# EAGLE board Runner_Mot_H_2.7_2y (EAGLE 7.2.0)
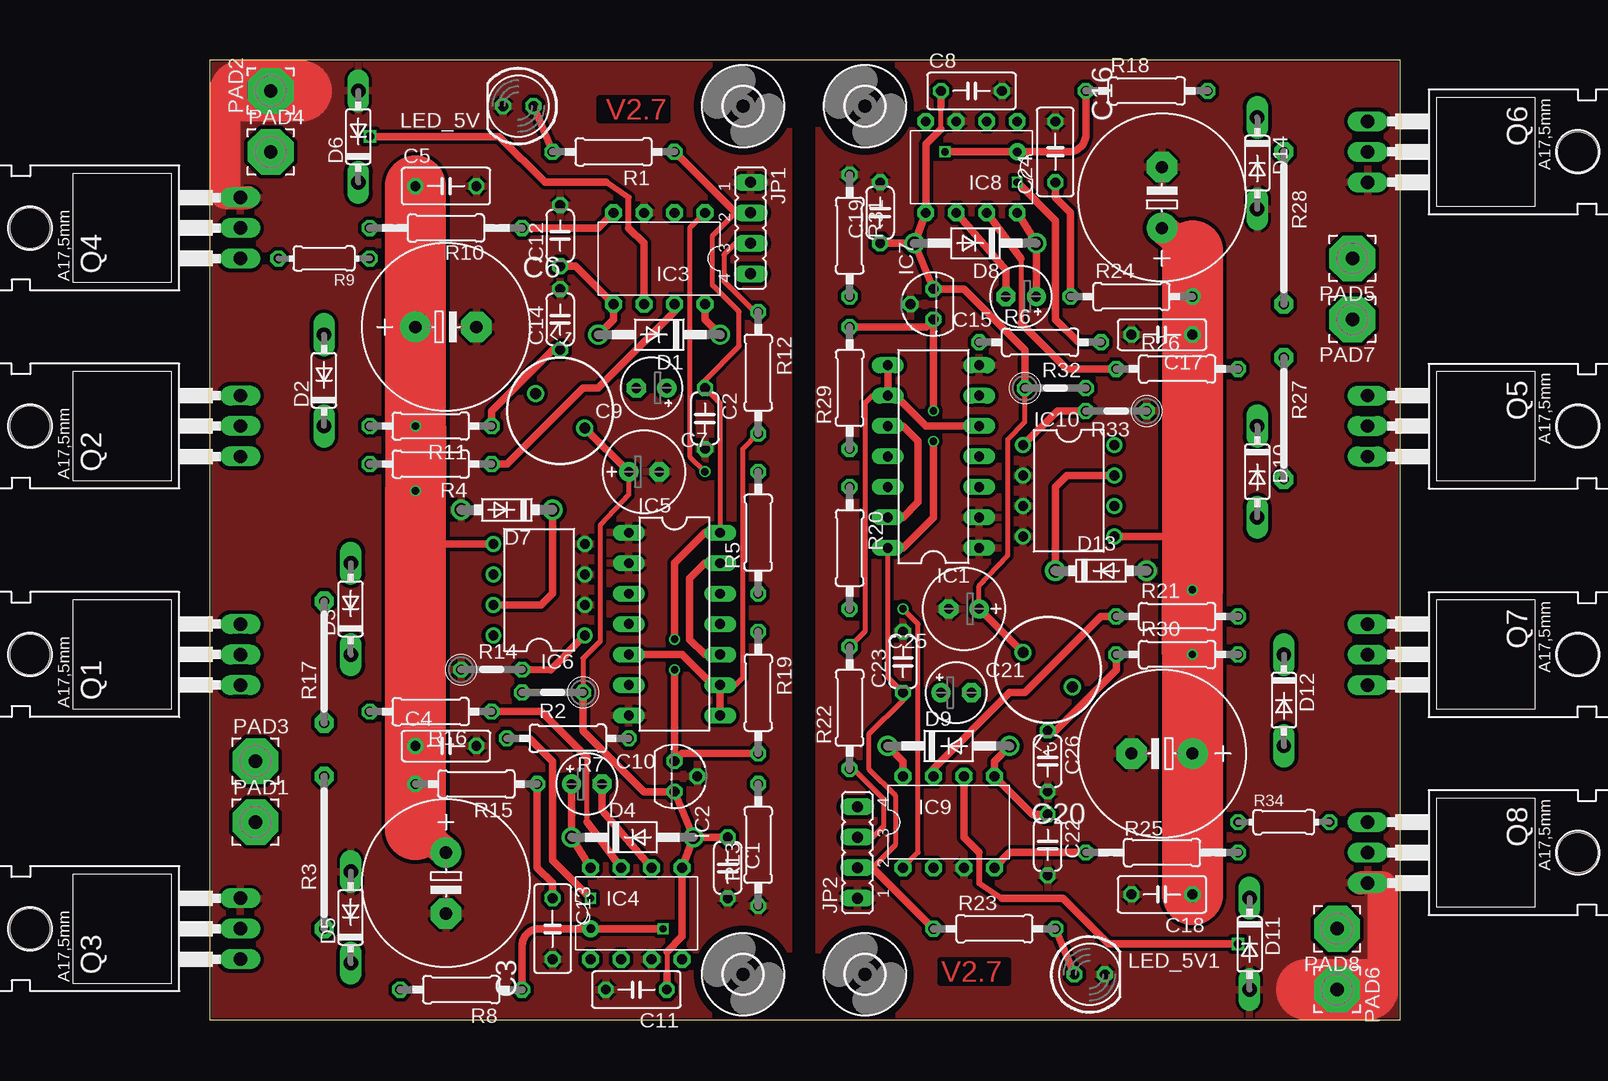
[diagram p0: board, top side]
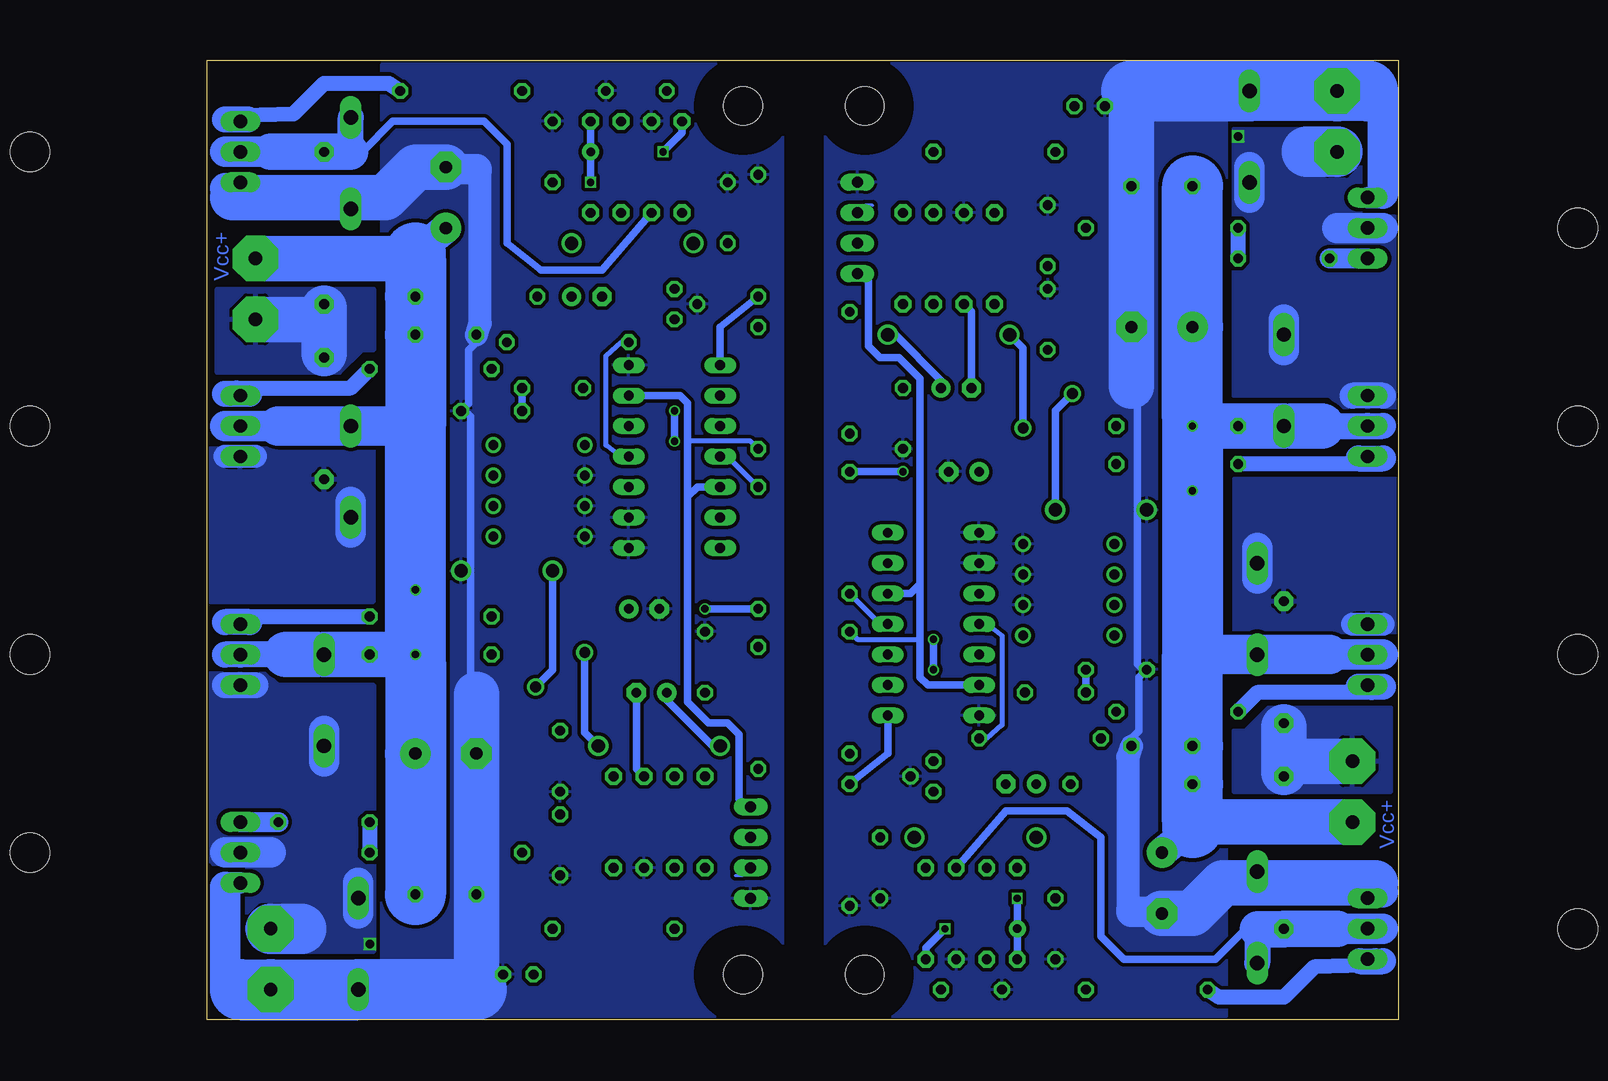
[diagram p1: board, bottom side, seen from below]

Size 99.26 x 80 mm. Coordinates in mm from the lower left corner, seen from the top.
Outline: 99.26,80 0,80 0,0 99.26,0 99.26,80
Copper layers (1*16): Top 0.035mm / dielectric 1.5mm / Bottom 0.035mm
Design rules "default *": minimum track width 6mil, minimum drill 12mil, track to track 12mil, track to pad 12mil, pad to pad 12mil, via to via 10mil, smd to smd 0mil, copper to edge 6mil, drill to drill 10mil, minimum pad ring 10mil, minimum via ring 6mil, stop-mask expansion 2mil, vias tented up to drill 100mil, thermal gap 10mil

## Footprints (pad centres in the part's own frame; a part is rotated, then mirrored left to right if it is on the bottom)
C050-024X044 = drill 0.813 octagon: 1 -2.54,0; 2 2.54,0
E5-13 = drill 1.016 pad 2.54: + -2.54,0 | drill 1.016 pad 2.54 octagon: - 2.54,0
C050-025X075 = drill 0.813 octagon: 1 -2.54,0; 2 2.54,0
C050-030X075 = drill 0.813 octagon: 1 -2.54,0; 2 2.54,0
E2,5-7 = drill 0.813 pad 1.6: + -1.27,0 | drill 0.813 pad 1.6 octagon: - 1.27,0
E2,5-5 = drill 0.813 pad 1.6: + -1.27,0 | drill 0.813 pad 1.6 octagon: - 1.27,0
DO41-10 = drill 1.118: A 5.08,0; C -5.08,0
DO35-7 = drill 1.2 long: A 3.81,0; C -3.81,0
DO41-7.6 = drill 1.1 pad 1.7: A 3.81,0; C -3.81,0
DIL14 = drill 0.813 long: 1 -7.62,-3.81; 2 -5.08,-3.81; 3 -2.54,-3.81; 4 0,-3.81; 5 2.54,-3.81; 6 5.08,-3.81; 7 7.62,-3.81; 8 7.62,3.81; 9 5.08,3.81; 10 2.54,3.81; 11 0,3.81; 12 -2.54,3.81; 13 -5.08,3.81; 14 -7.62,3.81
TO92 = drill 0.813 octagon: 1 -1.27,0; 2 0,1.905; 3 1.27,0
IRF_DIL08 = drill 0.813 pad 1.397 octagon: 1 -3.81,-3.81; 2 -1.27,-3.81; 3 1.27,-3.81; 4 3.81,-3.81; 5 3.81,3.81; 6 1.27,3.81; 7 -1.27,3.81; 8 -3.81,3.81
DIL08 = drill 0.813 pad 1.27: 1 -3.81,-3.81; 2 -1.27,-3.81; 3 1.27,-3.81; 4 3.81,-3.81; 5 3.81,3.81; 6 1.27,3.81; 7 -1.27,3.81; 8 -3.81,3.81
JP4 = drill 0.914 long: 1 -3.81,0; 2 -1.27,0; 3 1.27,0; 4 3.81,0
6000-XXXX-RC = drill 0.9 pad 1.422: 1 -2.5,0; 2 2.5,0
LED5MM = drill 0.813 octagon: A -1.27,0; K 1.27,0
3,81/1,1 = drill 1.118 pad 3.81 octagon: 1 0,0
TO220BH = drill 1.118 long: D 0,-6.35; G -2.54,-6.35; S 2.54,-6.35 | hole 3.302: 0,11.176
0207/10 = drill 0.813 octagon: 1 -5.08,0; 2 5.08,0
0207/5V = drill 0.813 octagon: 1 -2.54,0; 2 2.54,0
12 = drill 0.813 pad 1.6 octagon: 1 -6.35,0; 2 6.35,0
0204/7 = drill 0.813 octagon: 1 -3.81,0; 2 3.81,0
0207/12 = drill 0.813 octagon: 1 -6.35,0; 2 6.35,0
10 = drill 0.813 pad 1.6 octagon: 1 -5.08,0; 2 5.08,0
3,2 = hole 3.2: 0,0

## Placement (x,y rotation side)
C1  100nF  [C050-024X044]  43.18,12.69 270 top
C2  100nF  [C050-024X044]  41.27,50.16 270 top
C3  680u/50V  [E5-13]  19.68,11.42 270 top
C4  100nF  [C050-025X075]  19.68,22.85 0 top
C5  100nF  [C050-030X075]  19.68,69.52 0 top
C6  680u/50V  [E5-13]  19.68,57.77 0 top
C7  220u/16V  [E2,5-7]  36.19,45.71 0 top
C8  100nF  [C050-030X075]  63.5,77.46 0 top
C9  4u7  [E2,5-5]  36.83,52.7 180 top
C10  4u7  [E2,5-5]  31.43,19.67 0 top
C11  100nF  [C050-030X075]  35.56,2.53 180 top
C12  100nF  [C050-024X044]  29.21,65.39 90 top
C13  100nF  [C050-030X075]  28.58,7.61 270 top
C14  100nF  [C050-024X044]  29.21,58.41 90 top
C15  4u7  [E2,5-5]  67.63,60.32 180 top
C16  680u/50V  [E5-13]  79.38,68.57 90 top
C17  100nF  [C050-025X075]  79.38,57.14 180 top
C18  100nF  [C050-030X075]  79.38,10.47 180 top
C19  100nF  [C050-024X044]  55.88,67.3 90 top
C20  680u/50V  [E5-13]  79.38,22.21 180 top
C21  4u7  [E2,5-5]  62.23,27.29 0 top
C22  100nF  [C050-024X044]  69.85,14.6 270 top
C23  100nF  [C050-024X044]  57.78,29.83 90 top
C24  100nF  [C050-030X075]  70.48,72.38 90 top
C25  220u/16V  [E2,5-7]  62.87,34.28 180 top
C26  100nF  [C050-024X044]  69.85,21.58 270 top
D1  SF18G  [DO41-10]  37.47,57.14 180 top
D2  1.5KE51A  [DO35-7]  9.53,53.33 90 top
D3  1.5KE51A  [DO35-7]  11.75,34.28 90 top
D4  SF18G  [DO41-10]  35.24,15.23 0 top
D5  1.5KE51A  [DO35-7]  11.75,8.56 90 top
D6  1.5KE51A  [DO35-7]  12.38,73.65 90 top
D7  1N5819-T  [DO41-7.6]  24.77,42.54 180 top
D8  SF18G  [DO41-10]  63.82,64.76 180 top
D9  SF18G  [DO41-10]  61.59,22.85 0 top
D10  1.5KE51A  [DO35-7]  87.31,45.71 270 top
D11  1.5KE51A  [DO35-7]  86.68,6.34 270 top
D12  1.5KE51A  [DO35-7]  89.53,26.66 270 top
D13  1N5819-T  [DO41-7.6]  74.3,37.46 0 top
D14  1.5KE51A  [DO35-7]  87.31,71.43 270 top
IC1  4001N  [DIL14]  60.33,46.98 90 top
IC2  7805L  [TO92]  38.73,20.31 270 top
IC3  IRF_IR2184  [IRF_DIL08]  37.47,63.49 180 top
IC4  IRF_IR2184  [IRF_DIL08]  35.56,8.88 0 top
IC5  4001N  [DIL14]  38.73,33.01 270 top
IC6  LM2574N-ADJ  [DIL08]  27.45,35.87 90 top
IC7  7805L  [TO92]  60.33,59.68 90 top
IC8  IRF_IR2184  [IRF_DIL08]  63.5,71.11 180 top
IC9  IRF_IR2184  [IRF_DIL08]  61.59,16.5 0 top
IC10  LM2574N-ADJ  [DIL08]  71.61,44.12 270 top
JP1  PWM  [JP4]  45.09,66.03 270 top
JP2  PWM  [JP4]  53.98,13.96 90 top
L1  220uH  [6000-XXXX-RC]  29.21,50.79 325 top
L2  220uH  [6000-XXXX-RC]  69.85,29.2 145 top
LED_5V  Power  [LED5MM]  25.72,76.19 180 top
LED_5V1  Power  [LED5MM]  73.34,3.8 0 top
PAD1  36V-45V  [3,81/1,1]  3.81,16.5 0 top
PAD2  GND  [3,81/1,1]  5.08,77.46 90 top
PAD3  Motor_A  [3,81/1,1]  3.81,21.58 0 top
PAD4  Motor_B  [3,81/1,1]  5.08,72.38 0 top
PAD5  36V-45V  [3,81/1,1]  95.25,63.49 180 top
PAD6  GND  [3,81/1,1]  93.98,2.53 270 top
PAD7  Motor_A  [3,81/1,1]  95.25,58.41 180 top
PAD8  Motor_B  [3,81/1,1]  93.98,7.61 180 top
Q1  IRFB 4110  [TO220BH]  -3.81,30.47 90 top
Q2  IRFB 4110  [TO220BH]  -3.81,49.52 90 top
Q3  IRFB 4110  [TO220BH]  -3.81,7.61 90 top
Q4  IRFB 4110  [TO220BH]  -3.81,66.03 90 top
Q5  IRFB 4110  [TO220BH]  102.87,49.52 270 top
Q6  IRFB 4110  [TO220BH]  102.87,72.38 270 top
Q7  IRFB 4110  [TO220BH]  102.87,30.47 270 top
Q8  IRFB 4110  [TO220BH]  102.87,13.96 270 top
R1  1k8  [0207/10]  33.66,72.38 180 top
R2  18k  [0207/5V]  28.57,27.31 180 top
R3  0R  [12]  9.53,13.96 90 top
R4  4R7  [0207/10]  18.41,46.34 180 top
R5  4k7  [0207/10]  45.72,40.63 90 top
R6  4k7  [0207/10]  69.22,56.51 0 top
R7  4k7  [0207/10]  29.84,23.48 180 top
R8  4R7  [0207/10]  20.95,2.53 180 top
R9  4R7  [0204/7]  9.53,63.49 180 top
R10  4R7  [0207/12]  19.68,66.03 180 top
R11  0.47  [0207/10]  18.41,49.52 180 top
R12  4k7  [0207/10]  45.72,53.97 270 top
R13  100k  [0207/10]  45.72,14.6 90 top
R14  1k8  [0207/5V]  23.5,29.21 0 top
R15  0.47  [0207/10]  22.23,19.67 180 top
R16  4R7  [0207/10]  18.41,25.71 180 top
R17  0R  [10]  9.53,29.83 90 top
R18  4R7  [0207/10]  78.11,77.46 0 top
R19  100k  [0207/10]  45.72,27.29 270 top
R20  4k7  [0207/10]  53.34,39.36 270 top
R21  4R7  [0207/10]  80.64,33.65 0 top
R22  4k7  [0207/10]  53.34,26.02 90 top
R23  1k8  [0207/10]  65.41,7.61 0 top
R24  0.47  [0207/10]  76.83,60.32 0 top
R25  4R7  [0207/12]  79.38,13.96 0 top
R26  4R7  [0207/10]  80.64,54.28 0 top
R27  0R  [10]  89.53,50.16 270 top
R28  0R  [12]  89.53,66.03 270 top
R29  100k  [0207/10]  53.34,52.7 90 top
R30  0.47  [0207/10]  80.64,30.47 0 top
R31  100k  [0207/10]  53.34,65.39 270 top
R32  18k  [0207/5V]  70.48,52.68 0 top
R33  1k8  [0207/5V]  75.56,50.78 180 top
R34  4R7  [0204/7]  89.53,16.5 0 top
U$1  [3,2]  44.45,3.8 90 top
U$2  [3,2]  44.45,76.19 90 top
U$3  [3,2]  54.61,76.19 270 top
U$4  [3,2]  54.61,3.8 270 top

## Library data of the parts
C1-C26 L1 L2 R1 R2 R4-R16 R18-R26 R29-R34 = rcl
D1-D14 = diode
IC1 IC5 = 40xx
IC2 IC6 IC7 IC10 = linear
IC3 IC4 IC8 IC9 = AT3329-BTWS
JP1 JP2 R3 R17 R27 R28 = jumper
LED_5V LED_5V1 = led
PAD1-PAD8 = wirepad
Q1-Q8 = transistor-power
U$1-U$4 = holes

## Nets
GND: C1.2 C2.2 C3.- C4.2 C5.2 C6.- C7.- C11.2 C12.2 C13.2 C14.2 D5.A D6.A D7.A IC2.2 IC3.3 IC4.3 IC5.1 IC5.2 IC5.7 IC6.2 IC6.3 IC6.4 JP1.1 LED_5V.K PAD2.1 Q3.S Q4.S R13.1 R14.1
GND1: C8.2 C16.- C17.2 C18.2 C19.2 C20.- C22.2 C23.2 C24.2 C25.- C26.2 D11.A D13.A D14.A IC1.1 IC1.2 IC1.7 IC7.2 IC8.3 IC9.3 IC10.2 IC10.3 IC10.4 JP2.1 LED_5V1.K PAD6.1 Q6.S Q8.S R31.1 R33.1
N$1: IC3.1 R5.2
N$3: C10.- D5.C IC4.6 Q3.D R3.1
N$4: C10.+ D4.C IC4.8
N$5: IC4.7 R16.1
N$6: Q1.G R16.2
N$7: IC4.1 IC4.4 R7.2 R8.1
N$8: Q3.G R8.2
N$9: C9.- D2.A D6.C IC3.6 PAD4.1 Q2.S Q4.D
N$10: C9.+ D1.C IC3.8
N$11: IC3.7 R4.1
N$12: Q2.G R4.2
N$13: IC3.4 R10.1
N$14: Q4.G R9.2
N$15: C13.1 R15.1
N$16: C14.1 R11.1
N$17: IC5.4 R7.1
N$18: IC5.11 R5.1
N$19: IC5.6 IC5.12 JP1.4 R19.1
N$20: IC5.5 IC5.8 IC5.9 R12.2 R13.2
N$21: IC5.10 IC5.13
N$22: IC6.1 R2.2 R14.2
N$23: R9.1 R10.2
N$24: LED_5V.A R1.2
N$25: JP1.3 R12.1
N$27: PAD3.1 R3.2 R17.1
N$28: C15.+ D8.C IC8.8
N$29: D3.A Q1.S R17.2
N$30: IC8.7 R26.1
N$32: IC8.1 IC8.4 R6.2 R18.1
N$33: D7.C IC6.7 L1.1
N$34: Q6.G R18.2
N$35: C21.- D11.C D12.A IC9.6 PAD8.1 Q7.S Q8.D
N$36: C21.+ D9.C IC9.8
N$37: IC9.7 R21.1
N$38: Q7.G R21.2
N$39: IC1.4 R6.1
N$40: IC1.11 R20.1
N$41: IC1.6 IC1.12 JP2.4 R29.1
N$42: IC1.5 IC1.8 IC1.9 R22.2 R31.2
N$43: IC1.10 IC1.13
N$44: C15.- D14.C IC8.6 Q6.D R28.1
N$45: LED_5V1.A R23.2
N$46: IC9.1 R20.2
N$47: IC9.4 R25.1
N$48: JP2.3 R22.1
N$49: C24.1 R24.1
N$50: D10.A Q5.S R27.2
N$51: Q5.G R26.2
N$52: PAD7.1 R27.1 R28.2
N$53: C26.1 R30.1
N$54: IC10.1 R32.2 R33.2
N$55: D13.C IC10.7 L2.1
N$56: Q8.G R34.2
N$57: R25.2 R34.1
VCC1: C16.+ C17.1 C18.1 C20.+ D10.C D12.C IC10.5 PAD5.1 Q5.D Q7.D R24.2 R30.2
VCC2: C8.1 C19.1 C22.1 C25.+ D8.A D9.A IC7.3 IC8.5 IC9.5 L2.2 R32.1
VCC3: C23.1 IC1.14 IC7.1 JP2.2 R23.1 R29.2
VCC5: C2.1 IC2.1 IC5.14 JP1.2 R1.1 R19.2
VCC15: C1.1 C7.+ C11.1 C12.1 D1.A D4.A IC2.3 IC3.5 IC4.5 L1.2 R2.1
VCC24: C3.+ C4.1 C5.1 C6.+ D2.C D3.C IC6.5 PAD1.1 Q1.D Q2.D R11.2 R15.2

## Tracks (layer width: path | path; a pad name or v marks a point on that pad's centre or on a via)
GND
  Top 1.93: 1.27,68.57 3.17,68.57
  Top 2.54: 1.27,77.78 1.27,68.89
  Top 5.08: 2.54,77.46 7.62,77.46
  Bottom 0.61: 22.23,52.85 22.23,51.58 21.75,51.58 21.75,29.68 21.29,29.21 R14.1 21.59,28.58 21.59,24.12 22.23,23.48 C4.2 | 19.84,9.04 C3.-
  Bottom 1.27: 1.91,11.42 Q3.S 1.75,10.63
  Bottom 1.778: 1.75,10.63 1.91,10.63 | 1.27,68.57 Q4.S 1.91,68.57
  Bottom 1.93: C4.2 22.54,21.9 22.54,9.2 22.23,9.2 22.23,9.04
  Bottom 2.54: 1.91,10.63 1.27,10.63 | 22.23,9.04 19.84,9.04 | 1.27,68.89 1.27,77.46 2.54,77.46
  Bottom 3.81: 22.23,52.85 C6.- C5.2 22.23,77.46 | C3.- 17.14,8.88 14.61,11.42 1.91,11.42
  Bottom 5.08: 22.23,77.46 D6.A PAD2.1 2.54,77.46
  pour Bottom: 14.29,80 47.78,79.68 47.78,0.31 14.29,0.31
  pour Top: 0,-0.01 0,80 48.26,80 48.26,-0.01
GND1
  Top 1.93: 97.79,11.42 95.89,11.42
  Top 2.54: 97.79,2.21 97.79,11.1
  Top 5.08: 96.52,2.53 91.44,2.53
  Bottom 0.61: 76.83,27.14 76.83,28.41 77.31,28.41 77.31,50.31 77.78,50.78 R33.1 77.47,51.41 77.47,55.87 76.83,56.51 C17.2 | 79.22,70.95 C16.-
  Bottom 1.27: 97.16,68.57 Q6.S 97.31,69.36
  Bottom 1.778: 97.31,69.36 97.16,69.36 | 97.79,11.42 Q8.S 97.16,11.42
  Bottom 1.93: C17.2 76.52,58.09 76.52,70.79 76.83,70.79 76.83,70.95
  Bottom 2.54: 97.16,69.36 97.79,69.36 | 76.83,70.95 79.22,70.95 | 97.79,11.1 97.79,2.53 96.52,2.53
  Bottom 3.81: 76.83,27.14 C20.- C18.2 76.83,2.53 | C16.- 81.92,71.11 84.45,68.57 97.16,68.57
  Bottom 5.08: 76.83,2.53 D11.A PAD6.1 96.52,2.53
  pour Bottom: 84.77,-0.01 51.28,0.31 51.28,79.68 84.77,79.68
  pour Top: 99.06,80 99.06,-0.01 50.8,-0.01 50.8,80
N$1  (via drill 0.61)
  Top 0.406: v41.27,45.71 40.01,46.98 40.01,66.03 IC3.1
  Bottom 0.61: v41.27,45.71 R5.2
N$3
  Top 0.61: IC4.6 32.7,17.49 C10.-
  Bottom 0.152: D5.C 11.43,6.34 11.43,7.58
  Bottom 0.61: 11.68,7.58 12.73,7.58 15.24,5.07 22.86,5.07 24.77,6.98 24.77,15.23 27.62,17.45 32.7,17.45 IC4.6
  Bottom 2.184: 11.75,7.61 D5.C
  Bottom 2.54: 1.27,7.61 Q3.D 5.08,7.61
  Bottom 3.048: 5.08,7.61 R3.1 9.53,7.58 11.43,7.58 11.68,7.58
N$4
  Top 0.61: IC4.8 D4.C C10.+
N$5
  Top 0.406: 31.43,16.5 31.43,21.9
  Top 0.61: R16.1 27.62,25.71 31.43,21.9 | IC4.7 31.43,16.5
N$6
  Bottom 1.27: Q1.G 3.3,27.77 2.22,27.29 11.75,27.29 R16.2
  Bottom 2.184: 1.27,27.77 3.3,27.77
N$7  (via drill 0.6, 0.7 pad 1.42)
  Top 0.61: R8.1 26.04,6.19 arc-90 27.45,7.61 v31.75,7.61 v37.78,7.61 | R7.2 26.67,23.48 28.57,21.58 28.57,13.33 v31.75,10.15
  Bottom 0.61: v37.78,7.61 39.37,6.02 IC4.4 | IC4.1 v31.75,7.61 v31.75,10.15
N$8
  Bottom 0.152: 1.91,4.91 1.91,5.07 Q3.G
  Bottom 1.27: Q3.G 2.69,4.57 6.99,4.44 9.53,1.9 14.92,1.9 R8.2
  Bottom 2.184: 3.17,4.91 1.91,4.91 1.27,4.91
N$9  (via drill 0.7)
  Top 0.508: 34.92,66.03 34.92,68.57 33.02,69.84
  Top 0.61: 33.02,69.84 27.94,69.84 24.13,73.65 v13.34,73.65 | 34.92,66.03 36.2,64.76 IC3.6
  Bottom 0.61: C9.- 35.56,59.05 IC3.6
  Bottom 2.184: 1.27,52.06 3.81,52.06 | 1.27,66.03 3.81,66.03
  Bottom 2.54: 5.08,66.03 1.27,66.03 | 9.53,55.87 9.53,58.41 | 12.38,68.57 12.38,71.11
  Bottom 4.216: 7.62,72.38 PAD4.1
  pour Bottom: 0,51.11 4.6,51.11 5.71,52.06 13.65,52.06 13.65,74.28 3.81,74.28 3.17,73.65 3.17,66.98 0.32,66.98 0,66.66
N$10
  Top 0.61: IC3.8 41.27,58.41 D1.C
  Bottom 0.61: C9.+ 38.1,53.33 41.91,57.14 D1.C | C9.+
N$11
  Top 0.61: IC3.7 38.73,59.05 32.38,52.7 31.11,52.7 24.77,46.34 R4.1
N$12
  Bottom 0.457: Q2.G 1.43,46.98 3.3,46.82
  Bottom 1.27: Q2.G 2.54,46.34 R4.2
  Bottom 2.184: 3.3,46.82 1.27,46.82
N$13
  Top 0.61: R10.1 32.38,66.03 IC3.4
N$14
  Bottom 1.676: Q4.G R9.2
N$15
  Top 0.61: R15.1 27.3,12.69 28.57,11.42 C13.1
N$16
  Top 0.61: R11.1 23.5,50.79 28.57,55.87 C14.1
N$17
  Bottom 0.406: 34.29,33.01 33.02,32.06 33.02,24.6 34.29,23.48 R7.1
  Bottom 0.61: IC5.4 34.29,33.01
N$18
  Bottom 0.406: IC5.11 43.18,33.01 R5.1
N$19
  Bottom 0.406: 44.13,61.59 JP1.4 | R19.1 45.09,31.74 39.85,31.74
  Bottom 0.61: 44.13,61.59 44.13,56.19 43.18,55.23 41.59,55.23 39.85,53.49 39.85,36.34 | 39.85,36.34 40.64,35.55 IC5.12 43.18,35.55 | IC5.6 39.21,27.93 39.85,28.56 39.85,31.74 39.85,36.34
N$20
  Top 0.406: R12.2 44.45,47.62 44.45,28.56 43.81,27.93 IC5.9
  Top 0.61: IC5.8 IC5.9 41.91,27.93 39.37,30.47 IC5.5
  Bottom 0.61: R13.2 42.55,22.21 IC5.8
N$21
  Top 0.61: IC5.10 41.27,30.47 40.01,31.74 40.01,36.82 41.27,38.09 IC5.13
N$22
  Top 0.61: IC6.1 28.4,29.2 R14.2
  Bottom 0.254: R14.2
  Bottom 0.61: R14.2 R2.2
N$23
  Bottom 1.27: R9.1 R10.2
N$24
  Top 0.61: LED_5V.A R1.2
N$25
  Top 0.406: R12.1 45.4,59.05 42.86,61.59 42.86,63.81 43.81,64.76 JP1.3
N$27
  Bottom 0.152: R3.2 9.53,20.63 | 9.53,22.85 9.21,21.58 | R17.1 9.53,24.44
  Bottom 3.81: PAD3.1 9.21,21.58 | 9.53,20.63 9.53,22.85 9.53,24.44
  pour Bottom: 13.65,19.04 13.65,24.12 12.7,24.12 10.79,26.02 0.64,26.02 0.64,19.04
N$28
  Top 0.61: IC8.8 D8.C C15.+
N$29
  Bottom 1.93: 3.81,33.01 1.27,33.01
  Bottom 2.54: 11.75,36.82 11.75,39.36
  pour Bottom: 13.65,45.08 13.65,32.38 0,32.38 0,45.08
N$30
  Top 0.406: 67.63,63.49 67.63,58.09
  Top 0.61: R26.1 71.44,54.28 67.63,58.09 | IC8.7 67.63,63.49
N$32  (via drill 0.6, 0.7 pad 1.42)
  Top 0.61: R18.1 73.03,73.8 arc-90 71.61,72.38 v67.31,72.38 v61.28,72.38 | R6.2 72.39,56.51 70.48,58.41 70.48,66.66 v67.31,69.84
  Bottom 0.61: v61.28,72.38 59.69,73.97 IC8.4 | IC8.1 v67.31,72.38 v67.31,69.84
N$33
  Top 0.61: D7.C 28.57,35.55 27.62,34.6 IC6.7
  Bottom 0.61: D7.C 28.57,50.81 L1.1
N$34
  Bottom 0.152: 97.16,75.08 97.16,74.92 Q6.G
  Bottom 1.27: Q6.G 96.37,75.42 92.08,75.55 89.53,78.09 84.14,78.09 R18.2
  Bottom 2.184: 95.89,75.08 97.16,75.08 97.79,75.08
N$35  (via drill 0.7)
  Top 0.508: 64.14,13.96 64.14,11.42 66.04,10.15
  Top 0.61: 66.04,10.15 71.12,10.15 74.93,6.34 v85.72,6.34 | 64.14,13.96 62.87,15.23 IC9.6
  Bottom 0.61: C21.- 63.5,20.94 IC9.6
  Bottom 2.184: 97.79,27.93 95.25,27.93 | 97.79,13.96 95.25,13.96
  Bottom 2.54: 93.98,13.96 97.79,13.96 | 89.53,24.12 89.53,21.58 | 86.68,11.42 86.68,8.88
  Bottom 4.216: 91.44,7.61 PAD8.1
  pour Bottom: 99.06,28.88 94.46,28.88 93.34,27.93 85.41,27.93 85.41,5.71 95.25,5.71 95.89,6.34 95.89,13.01 98.74,13.01 99.06,13.33
N$36
  Top 0.61: IC9.8 57.78,21.58 D9.C
  Bottom 0.61: C21.+ 60.96,26.66 57.15,22.85 D9.C | C21.+
N$37
  Top 0.61: IC9.7 60.33,20.94 66.67,27.29 67.94,27.29 74.3,33.65 R21.1
N$38
  Bottom 0.457: Q7.G 97.63,33.01 95.76,33.17
  Bottom 1.27: Q7.G 96.52,33.65 R21.2
  Bottom 2.184: 95.76,33.17 97.79,33.17
N$39
  Bottom 0.406: 64.77,46.98 66.04,47.93 66.04,55.39 64.77,56.51 R6.1
  Bottom 0.61: IC1.4 64.77,46.98
N$40
  Bottom 0.406: IC1.11 55.88,46.98 R20.1
N$41
  Bottom 0.406: 54.93,18.4 JP2.4 | R29.1 53.98,48.25 59.21,48.25
  Bottom 0.61: 54.93,18.4 54.93,23.8 55.88,24.75 57.47,24.75 59.21,26.5 59.21,43.65 | 59.21,43.65 58.42,44.44 IC1.12 55.88,44.44 | IC1.6 59.85,52.06 59.21,51.43 59.21,48.25 59.21,43.65
N$42
  Top 0.406: R22.2 54.61,32.38 54.61,51.43 55.24,52.06 IC1.9
  Top 0.61: IC1.8 IC1.9 57.15,52.06 59.69,49.52 IC1.5
  Bottom 0.61: R31.2 56.52,57.77 IC1.8
N$43
  Top 0.61: IC1.10 57.78,49.52 59.05,48.25 59.05,43.17 57.78,41.9 IC1.13
N$44
  Top 0.61: IC8.6 66.36,62.5 C15.-
  Bottom 0.152: D14.C 87.63,73.65 87.63,72.41
  Bottom 0.61: 87.38,72.41 86.33,72.41 83.82,74.92 76.2,74.92 74.3,73.02 74.3,64.76 71.44,62.54 66.36,62.54 IC8.6
  Bottom 2.184: 87.31,72.38 D14.C
  Bottom 2.54: 97.79,72.38 Q6.D 93.98,72.38
  Bottom 3.048: 93.98,72.38 R28.1 89.53,72.41 87.63,72.41 87.38,72.41
N$45
  Top 0.61: LED_5V1.A R23.2
N$46  (via drill 0.61)
  Top 0.406: v57.78,34.28 59.05,33.01 59.05,13.96 IC9.1
  Bottom 0.61: v57.78,34.28 R20.2
N$47
  Top 0.61: R25.1 66.67,13.96 IC9.4
N$48
  Top 0.406: R22.1 53.66,20.94 56.2,18.4 56.2,16.18 55.24,15.23 JP2.3
N$49
  Top 0.61: R24.1 71.75,67.3 70.48,68.57 C24.1
N$50
  Bottom 1.93: 95.25,46.98 97.79,46.98
  Bottom 2.54: 87.31,43.17 87.31,40.63
  pour Bottom: 85.41,34.91 85.41,47.62 99.06,47.62 99.06,34.91
N$51
  Bottom 1.27: Q5.G 95.76,52.22 96.84,52.7 87.31,52.7 R26.2
  Bottom 2.184: 97.79,52.22 95.76,52.22
N$52
  Bottom 0.152: R28.2 89.53,59.36 | 89.53,57.14 89.85,58.41 | R27.1 89.53,55.55
  Bottom 3.81: PAD7.1 89.85,58.41 | 89.53,59.36 89.53,57.14 89.53,55.55
  pour Bottom: 85.41,60.95 85.41,55.87 86.36,55.87 88.27,53.97 98.42,53.97 98.42,60.95
N$53
  Top 0.61: R30.1 75.56,29.2 70.48,24.12 C26.1
N$54
  Top 0.61: IC10.1 70.66,50.79 R33.2
  Bottom 0.254: R33.2
  Bottom 0.61: R33.2 R32.2
N$55
  Top 0.61: D13.C 70.48,44.44 71.44,45.39 IC10.7
  Bottom 0.61: D13.C 70.48,29.18 L2.1
N$56
  Bottom 1.676: Q8.G R34.2
N$57
  Bottom 1.27: R34.1 R25.2
VCC1  (via drill 0.61)
  Top 0.406: v81.92,35.87 80.01,35.23
  Top 0.61: 80.01,35.23 v81.91,35.87 | 81.28,64.44 81.28,64.76 81.92,64.12 | IC10.5 81.92,40.31
  Top 2.54: 81.28,64.44 C16.+
  Top 5.08: 81.92,64.12 81.92,40.31 v81.92,35.87 v81.92,30.47 C18.1
  Bottom 0.254: C18.1 81.92,10.15 | 81.92,40.63 83.19,40
  Bottom 0.406: 81.92,40.63 81.91,40.47
  Bottom 0.61: 81.91,49.36 81.92,49.52
  Bottom 2.184: 97.79,30.47 Q7.D 92.71,30.47 | D12.C 90.17,30.47
  Bottom 2.54: 81.92,63.97 C16.+ | v81.92,30.47 81.92,29.83 | 97.79,49.52 Q5.D 93.34,49.52
  Bottom 3.302: 81.92,49.52 D10.C 93.34,49.52
  Bottom 3.81: v81.92,30.47 R30.2 D12.C | PAD5.1 81.92,63.49 | 92.71,30.47 90.17,30.47
  Bottom 5.08: 81.92,63.97 81.92,63.49 R24.2 C17.1 81.92,49.52 | 81.92,29.83 C20.+ C18.1 | 81.91,49.36 81.91,40.47 81.91,35.55 | v81.92,30.47 v81.92,35.87
VCC2
  Top 0.406: 60.96,74.28 60.96,76.19 | C25.+ 64.14,36.19 66.52,38.73 66.52,48.41 67.94,49.84 R32.1
  Top 0.61: D8.A IC7.3 62.87,60.95 67.94,55.87 R32.1 | 60.96,76.19 C8.1 | 60.96,74.28 59.69,73.02 IC8.5 D8.A | D9.A 65.41,21.58 IC9.5 68.58,17.13 C22.1 | C19.1 D8.A | C25.+ 64.16,34.28 L2.2
  Bottom 0.61: L2.2 67.8,23.98 D9.A
VCC3  (via drill 0.6)
  Top 0.254: C23.1
  Top 0.406: IC1.14 56.52,28.56 C23.1 57.78,26.66 54.93,23.8 54.93,20.94 57.15,18.72 57.15,14.6 55.24,12.69
  Top 0.61: R23.1 55.24,12.69 JP2.2 | IC1.14 57.78,39.36 60.33,41.9 v60.33,48.25 | v60.33,50.79 IC7.1 59.69,57.77 R29.2
  Bottom 0.254: JP2.2 54.61,12.05 55.24,12.05
  Bottom 0.61: v60.33,48.25 v60.33,50.79
VCC5  (via drill 0.6)
  Top 0.254: C2.1
  Top 0.406: IC5.14 42.55,51.43 C2.1 41.27,53.33 44.13,56.19 44.13,59.05 41.91,61.27 41.91,65.39 43.81,67.3
  Top 0.61: R1.1 43.81,67.3 JP1.2 | IC5.14 41.27,40.63 38.73,38.09 v38.73,31.74 | v38.73,29.2 IC2.1 39.37,22.21 R19.2
  Bottom 0.254: JP1.2 44.45,67.93 43.81,67.93
  Bottom 0.61: v38.73,31.74 v38.73,29.2
VCC15
  Top 0.406: 38.1,5.71 38.1,3.8 | C7.+ 34.92,43.8 32.54,41.27 32.54,31.58 31.11,30.15 R2.1
  Top 0.61: D4.A IC2.3 36.2,19.04 31.11,24.12 R2.1 | 38.1,3.8 C11.1 | 38.1,5.71 39.37,6.98 IC4.5 D4.A | D1.A 33.66,58.41 IC3.5 30.48,62.86 C12.1 | C1.1 D4.A | C7.+ 34.91,45.71 L1.2
  Bottom 0.61: L1.2 31.26,56.01 D1.A
VCC24  (via drill 0.61)
  Top 0.406: v17.14,44.12 19.05,44.76
  Top 0.61: 19.05,44.76 v17.15,44.12 | 17.78,15.55 17.78,15.23 17.14,15.87 | IC6.5 17.14,39.68
  Top 2.54: 17.78,15.55 C3.+
  Top 5.08: 17.14,15.87 17.14,39.68 v17.14,44.12 v17.14,49.52 C5.1
  Bottom 0.254: C5.1 17.14,69.84 | 17.14,39.36 15.88,40
  Bottom 0.406: 17.14,39.36 17.15,39.52
  Bottom 0.61: 17.15,30.63 17.14,30.47
  Bottom 2.184: 1.27,49.52 Q2.D 6.35,49.52 | D2.C 8.89,49.52
  Bottom 2.54: 17.14,16.02 C3.+ | v17.14,49.52 17.14,50.16 | 1.27,30.47 Q1.D 5.71,30.47
  Bottom 3.302: 17.14,30.47 D3.C 5.71,30.47
  Bottom 3.81: v17.14,49.52 R11.2 D2.C | PAD1.1 17.14,16.5 | 6.35,49.52 8.89,49.52
  Bottom 5.08: 17.14,16.02 17.14,16.5 R15.2 C4.1 17.14,30.47 | 17.14,50.16 C6.+ C5.1 | 17.15,30.63 17.15,39.52 17.15,44.44 | v17.14,49.52 v17.14,44.12

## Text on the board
Top: V2.7 | V2.7
Bottom: Vcc+ | Vcc+
Unrouted: Do not use to produce a PCB! | Do not use to produce a PCB! | Do not use to produce a PCB! | Do not use to produce a PCB!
